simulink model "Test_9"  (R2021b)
settings: Solver=VariableStepAuto  StartTime=0.0  StopTime=180  MaxStep=1/(50*80)
undefined symbols (not defined in the file): Ion, Lithium
libraries: fl_lib x6, nesl_utility x5, spsRMSLib x2, ee_lib x2, spsBatteryLib x1, spsCurrentVoltageSimscapeInterfaceLib x1, simulink x1, spspowerguiLib x1

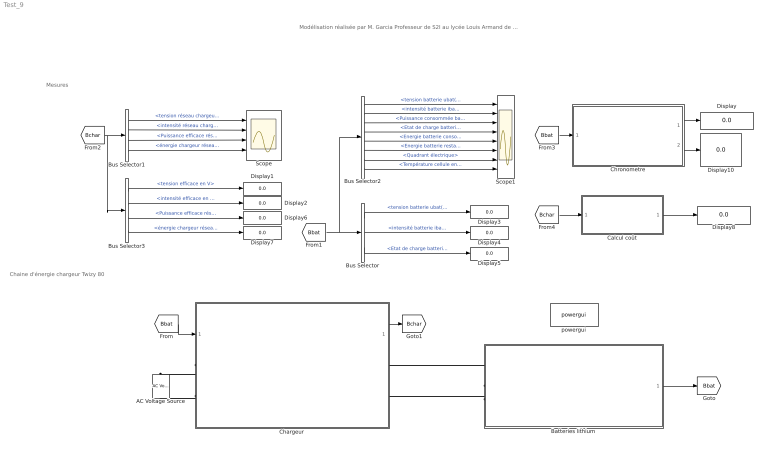
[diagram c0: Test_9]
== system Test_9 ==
  note: Mesures
  note: Chaine d'énergie chargeur Twizy 80
  note: Modélisation réalisée par M. Garcia Professeur de S2I au lycée Louis Armand de Nogent sur Marne
  AC Voltage Source : fl_lib/Electrical/Electrical Sources/AC Voltage Source  amp=230*sqrt(2) V  shift=0 deg  frequency=50 Hz  omega=0 rad/s
  Batteries lithium : Subsystem  mask{Ubat_n=54, Qbat_n=105, Soc_init=10, Soc_min=10, T_amb=35, T_init=35, Nb_cycles=1000, Nb_charge_mensuelle=20, Nb_mois=0}
      mask prompts: Ubat_n "Tension nominale batterie en V"; Qbat_n "Capacité nominale en A.h"; Soc_init "Etat de charge initial"; Soc_min "Seuil minimum en %"; T_amb "Température ambiante extérieure en °C"; T_init "Température initiale du bloc batteries en °C"; Nb_cycles "Durée de vie batterie en nombre de cycles"; Nb_charge_mensuelle "Nombre de recharges mensuelles"; Nb_mois "Nombre de mois d'utilisation"
  Bus Selector : BusSelector  OutputSignals=tension batterie ubat(t),intensité batterie ibat(t),Etat de charge batterie soc(t) en %
  Bus Selector1 : BusSelector  OutputSignals=tension réseau chargeur en V,intensité réseau chargeur en A,Puissance efficace réseau chargeur en W,énergie chargeur réseau en Wh
  Bus Selector2 : BusSelector  OutputSignals=tension batterie ubat(t),intensité batterie ibat(t),Puissance consommée batterie pbat(t) en W,Etat de charge batterie soc(t) en %,Energie batterie consommée wbat_cons(t) en Wh,Energie batterie restante wbat_rest(t) en Wh,Quadrant électrique,Température cellule en °C
  Bus Selector3 : BusSelector  OutputSignals=tension efficace en V,intensité efficace en A,Puissance efficace réseau chargeur en W,énergie chargeur réseau en Wh
  Calcul coût : Subsystem  mask{P_Hc=0.1243}
      mask prompts: P_Hc "Coût du kWh en € TTC"
  Chargeur : Subsystem  mask{Imax=30, rend_charg=94, Fp_charg=0.9, Long=3.75, Se=2.5}
      mask prompts: Imax "Intensité maximale de charge en A"; rend_charg "Rendement chargeur en %"; Fp_charg "Facteur de puissance chargeur"; Long "Longueur câble en m"; Se "Section câble en mm²"
  Chronometre : Subsystem
  Display{,1..8,10} (10 alike) : Display
  Scope : Scope  NumInputPorts=4
  Scope1 : Scope  NumInputPorts=8
  powergui : spspowerguiLib/powergui  Priority=1  SimulationMode=Discrete  SampleTime=0.1  frequency=60  Iterations=50  frequencyindice=0  Pbase=100e6  ErrMax=1e-4  UnitsV=kV  UnitsW=MW  buscounter=0  FunctionMessages=off  echomessages=off  EnableUseOfTLC=off  CurrentSourceSwitches=off  DisableSnubberDevices=off  DisableRonSwitches=off  DisableVfSwitches=off  DisplayEquations=off  AutomaticDiscreteSolvers=on  SolverType=Tustin/Backward Euler (TBE)  Interpol=off  ExternalGateDelay=off  methode=off  Ts=100  x0status=blocks  SPID=on  SwTol=0  HookPort=off  NonlinearTolerance=1e-4  nMaxIteration=100  ContinueOnMaxIteration=off  RestoreLinks=warning  ResistiveCurrentMeasurement=off  Frange=[0:2:500]  Ylog=off  Xlog=on  ShowGrid=off  save=off  variable=ZData  structure=0  ZoomFFT=off  StartTime=0.0  cycles=1  DisplayStyle=1  fundamental=60  FreqAxis=off  MaxFrequency=1000  frequencyindicesteady=1  RmsSteady=1  display=off
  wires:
  Bus Selector/2 -> Display4/1  "<intensité batterie ibat(t)>"
  [Bbat] -> Bus Selector2/1, Bus Selector/1
  Bus Selector2/1 -> Scope1/1  "<tension batterie ubat(t)>"
  Bus Selector2/2 -> Scope1/2  "<intensité batterie ibat(t)>"
  Bus Selector2/3 -> Scope1/3  "<Puissance consommée batterie pbat(t) en W>"
  Bus Selector/1 -> Display3/1  "<tension batterie ubat(t)>"
  Bus Selector/3 -> Display5/1  "<Etat de charge batterie soc(t) en %>"
  Batteries lithium/1(Bus batterie) -> [Bbat]
  Bus Selector2/4 -> Scope1/4  "<Etat de charge batterie soc(t) en %>"
  Bus Selector2/7 -> Scope1/7  "<Quadrant électrique>"
  Bus Selector2/5 -> Scope1/5  "<Energie batterie consommée wbat_cons(t) en Wh>"
  Bus Selector2/6 -> Scope1/6  "<Energie batterie restante wbat_rest(t) en Wh>"
  [Bbat] -> Chargeur/1(bus_bat)
  Chargeur/1(Bus_chargeur) -> [Bchar]
  [Bchar] -> Bus Selector3/1, Bus Selector1/1
  Bus Selector1/1 -> Scope/1  "<tension réseau chargeur en V>"
  Bus Selector1/2 -> Scope/2  "<intensité réseau chargeur en A>"
  Bus Selector1/3 -> Scope/3  "<Puissance efficace réseau chargeur en W>"
  Bus Selector1/4 -> Scope/4  "<énergie chargeur réseau en Wh>"
  Bus Selector3/1 -> Display1/1  "<tension efficace en V>"
  Bus Selector3/2 -> Display2/1  "<intensité efficace en A>"
  Bus Selector3/3 -> Display6/1  "<Puissance efficace réseau chargeur en W>"
  Bus Selector3/4 -> Display7/1  "<énergie chargeur réseau en Wh>"
  [Bbat] -> Chronometre/1(Bus Batterie)
  [Bchar] -> Calcul coût/1(Bus chargeur)
  Calcul coût/1(Cout en €) -> Display8/1
  Chronometre/2(Mesure temps de charge HH mm ss) -> Display10/1
  Chronometre/1(Mesure temps de charge h) -> Display/1
  Bus Selector2/8 -> Scope1/8  "<Température cellule en °C>"
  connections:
  Batteries lithium/LConn1 -- Chargeur/RConn1
  Batteries lithium/LConn2 -- Chargeur/RConn2
  Chargeur/LConn2 -- AC Voltage Source/RConn1
  Chargeur/LConn1 -- AC Voltage Source/LConn1

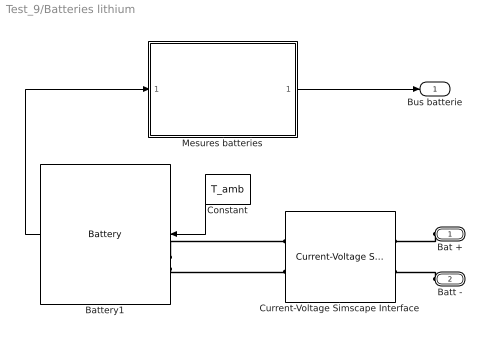
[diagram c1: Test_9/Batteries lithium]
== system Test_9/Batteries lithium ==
  Battery1 : spsBatteryLib/Battery  BatType=Lithium-Ion  ShowTempParam=on  ThermalPreset=no  ShowAgeParam=on  NomV=Ubat_n  NomQ=Qbat_n  SOC=Soc_init  Batt_Tr=30  PresetModel=on  MaxQ=105  MinV=40.5  FullV=62.8553  Dis_rate=45.6522  R=0.0051429  Normal_OP=94.9565  expZone="[58.3408       5.1587]"  current=[100 150 200]  Units=Time  Tci=T_init  NomT=25  T2=0  MaxQ2=Qbat_n/1.1517  FullV2=1.1933*Ubat_n  Normal_OP2=Ubat_n/1.1576  expZone2=[1.1338*Ubat_n Qbat_n/61]  Rca=0.06  ti=1000  Dp=0  Neq0=Nb_charge_mensuelle*Nb_mois  Tsim=30  Ta1=23  Qeol=0.9*Qbat_n  Reol=0.0126*1.2  Char_age=[0.38*Qbat_n, 0.495*Qbat_n]  Dis_age=[0.38*Qbat_n, 2*Qbat_n]  N1=Nb_cycles  N2=7*Nb_cycles  N3=Nb_cycles/1.5  N4=Nb_cycles*0.9733  Ta2=45  N5=Nb_cycles*0.655
  Constant : Constant  Value=T_amb
  Current-Voltage Simscape Interface : spsCurrentVoltageSimscapeInterfaceLib/Current-Voltage Simscape Interface  DFT=off  FMode=Unit delay (discrete)  T=1e-6  Ts=-1  i0=0  v0=52  Sd=Simscape side  Measurements=off
  Mesures batteries : Subsystem
  Bat + : PMIOPort  Side=Left
  Batt - : PMIOPort  Port=2  Side=Left
  Bus batterie : Outport  VectorParamsAs1DForOutWhenUnconnected=off
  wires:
  Battery1/1 -> Mesures batteries/1(Bus batteries)
  Mesures batteries/1(Bus_ batteries) -> Bus batterie/1
  Constant/1 -> Battery1/1
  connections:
  Battery1/LConn2 -- Current-Voltage Simscape Interface/LConn2
  Battery1/LConn1 -- Current-Voltage Simscape Interface/LConn1
  Bat +/RConn1 -- Current-Voltage Simscape Interface/RConn1
  Batt -/RConn1 -- Current-Voltage Simscape Interface/RConn2

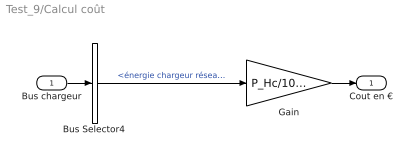
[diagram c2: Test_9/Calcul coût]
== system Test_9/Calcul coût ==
  Bus chargeur : Inport
  Bus Selector4 : BusSelector  OutputSignals=énergie chargeur réseau en Wh
  Gain : Gain  Gain=P_Hc/1000
  Cout en € : Outport  VectorParamsAs1DForOutWhenUnconnected=off
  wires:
  Bus Selector4/1 -> Gain/1  "<énergie chargeur réseau en Wh>"
  Gain/1 -> Cout en €/1
  Bus chargeur/1 -> Bus Selector4/1

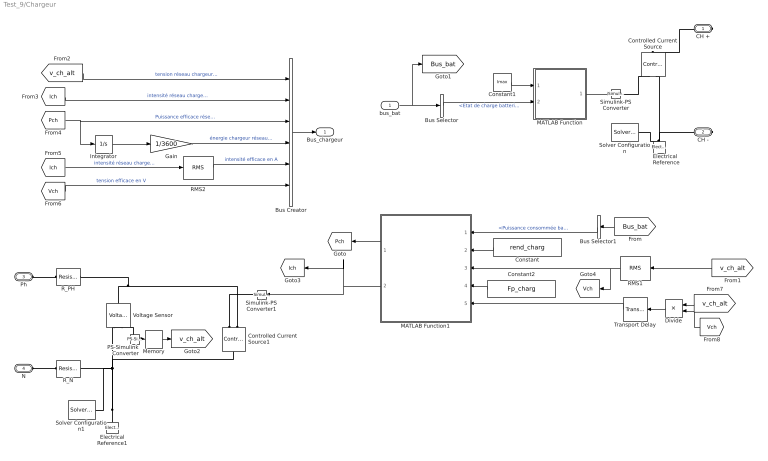
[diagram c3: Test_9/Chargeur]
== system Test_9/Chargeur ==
  bus_bat : Inport
  Bus Creator : BusCreator  Inputs=6
  Bus Selector : BusSelector  OutputSignals=Etat de charge batterie soc(t) en %
  Bus Selector1 : BusSelector  OutputSignals=Puissance consommée batterie pbat(t) en W
  Constant : Constant  Value=rend_charg
  Constant1 : Constant  Value=Imax
  Constant2 : Constant  Value=Fp_charg
  Controlled Current Source : fl_lib/Electrical/Electrical Sources/Controlled Current Source
  Controlled Current Source1 : fl_lib/Electrical/Electrical Sources/Controlled Current Source
  Divide : Product  Inputs=*/
  Electrical Reference : fl_lib/Electrical/Electrical Elements/Electrical Reference
  Electrical Reference1 : fl_lib/Electrical/Electrical Elements/Electrical Reference
  Gain : Gain  Gain=1/3600
  Integrator : Integrator
  MATLAB Function : MATLAB Function  TreatAsAtomicUnit=on
  MATLAB Function1 : MATLAB Function  TreatAsAtomicUnit=on
  Memory : Memory  LinearizeMemory=on
  PS-Simulink Converter : nesl_utility/PS-Simulink Converter  PhysicalDomain=network_engine_domain  SubClassName=ps_output  LeftPortType=input  RightPortType=output  PseudoPeriodic=off  Frequencies=[]  Unit=1  AffineConversion=off
  RMS1 : spsRMSLib/RMS  TrueRMS=on  Freq=50  RMSInit=230  Ts=0
  RMS2 : spsRMSLib/RMS  TrueRMS=on  Freq=50  RMSInit=0  Ts=0
  R_N : ee_lib/Passive/Resistor  R=Long*22e-3/Se Ohm  R_tol=5  enable_R_tol=0  tol_distribution=1  nSigma=4  enable_operating_limits=0  operating_limit_action=2  max_working_voltage=100 V  power_rating=1 W  enable_faults=0  fault_action=1  R_faulted=inf Ohm  enable_temporal_fault=0  t_fault=1 s  enable_behavioral_fault=0  max_permissible_current=1 A  t_fail_on_current=1 s  noise_mode=0  sample_time=1e-3 s  repeatability=1  auto_seed=676943032  user_seed=0  Tdevice=25 degC  power_derating_T1=70 degC  power_derating_T2=155 degC  operating_temperature_range_vec=[-50, 150] degC  alpha=3.93e-3 1/K  Tmeas=25 degC  thermal_mass=100 J/K  temperature_specify=off  temperature_priority=High  temperature=298.15 K  temperature_nominal_specify=off  temperature_nominal_unit=K  temperature_nominal_value=1
  R_PH : ee_lib/Passive/Resistor  R=Long*22e-3/Se Ohm  R_tol=5  enable_R_tol=0  tol_distribution=1  nSigma=4  enable_operating_limits=0  operating_limit_action=2  max_working_voltage=100 V  power_rating=1 W  enable_faults=0  fault_action=1  R_faulted=inf Ohm  enable_temporal_fault=0  t_fault=1 s  enable_behavioral_fault=0  max_permissible_current=1 A  t_fail_on_current=1 s  noise_mode=0  sample_time=1e-3 s  repeatability=1  auto_seed=4168664255  user_seed=0  Tdevice=25 degC  power_derating_T1=70 degC  power_derating_T2=155 degC  operating_temperature_range_vec=[-50, 150] degC  alpha=3.93e-3 1/K  Tmeas=25 degC  thermal_mass=100 J/K  temperature_specify=off  temperature_priority=High  temperature=298.15 K  temperature_nominal_specify=off  temperature_nominal_unit=K  temperature_nominal_value=1
  Simulink-PS Converter : nesl_utility/Simulink-PS Converter  PhysicalDomain=network_engine_domain  SubClassName=ps_input  LeftPortType=input  RightPortType=output  PseudoPeriodic=off  Frequencies=[]  NoiseDistribution=none  NoiseParameters=[]  Unit=A  AffineConversion=off  FilteringAndDerivatives=provide  SimscapeFilterOrder=1  InputFilterTimeConstant=0.001  UdotUserProvided=0
  Simulink-PS Converter1 : nesl_utility/Simulink-PS Converter  PhysicalDomain=network_engine_domain  SubClassName=ps_input  LeftPortType=input  RightPortType=output  PseudoPeriodic=off  Frequencies=[]  NoiseDistribution=none  NoiseParameters=[]  Unit=1  AffineConversion=off  FilteringAndDerivatives=provide  SimscapeFilterOrder=1  InputFilterTimeConstant=0.001  UdotUserProvided=0
  Solver Configuration : nesl_utility/Solver Configuration  PhysicalDomain=network_engine_domain  SubClassName=solver  LeftPortType=input  RightPortType=generic  Tones=[]  Harmonics=[]  SimulateNoise=off  Profile=off  UseLocalSampling=off  EnableSwitchedLinearOptims=on  FrequencyDomain=off  UseCCode=off  RelTol=0.001  AbsTol=1e-06  MinStep=1e-09  ToWorkspace=off  RevertToSquareIcSolve=off  NumHomotopyIterations=100  PhasorMode=off  PhasorModeNumHarmonics=1  DoDC=off  ResidualTolerance=1e-09  UseLocalSolver=off  LocalSolverChoice=NE_BACKWARD_EULER_ADVANCER  LocalSolverSampleTime=0.01  DoFixedCost=off  MaxNonlinIter=3  MaxModeIter=2  ComputeImpulses=off  ImpulseIterations=2  LinearAlgebra=auto  EquationFormulation=NE_TIME_EF  DelaysMemoryBudget=1024  AutomaticFiltering=on  FilteringTimeConstant=0.001  PartitionStorageMethod=AS_NEEDED  PartitionMemoryBudget=1024  PartitionMethod=FAST
  Solver Configuration1 : nesl_utility/Solver Configuration  PhysicalDomain=network_engine_domain  SubClassName=solver  LeftPortType=input  RightPortType=generic  Tones=[]  Harmonics=[]  SimulateNoise=off  Profile=off  UseLocalSampling=off  EnableSwitchedLinearOptims=on  FrequencyDomain=off  UseCCode=off  RelTol=0.001  AbsTol=1e-06  MinStep=1e-09  ToWorkspace=off  RevertToSquareIcSolve=off  NumHomotopyIterations=100  PhasorMode=off  PhasorModeNumHarmonics=1  DoDC=off  ResidualTolerance=1e-09  UseLocalSolver=off  LocalSolverChoice=NE_BACKWARD_EULER_ADVANCER  LocalSolverSampleTime=0.001  DoFixedCost=off  MaxNonlinIter=3  MaxModeIter=2  ComputeImpulses=off  ImpulseIterations=2  LinearAlgebra=auto  EquationFormulation=NE_TIME_EF  DelaysMemoryBudget=1024  AutomaticFiltering=on  FilteringTimeConstant=0.001  PartitionStorageMethod=AS_NEEDED  PartitionMemoryBudget=1024  PartitionMethod=FAST
  Transport Delay : TransportDelay  DelayTime=acos(Fp_charg)*0.02/(2*pi)
  Voltage Sensor : fl_lib/Electrical/Electrical Sensors/Voltage Sensor
  CH + : PMIOPort  Side=Right
  CH - : PMIOPort  Port=2  Side=Right
  Ph : PMIOPort  Port=3  Side=Left
  N : PMIOPort  Port=4  Side=Left
  Bus_chargeur : Outport  VectorParamsAs1DForOutWhenUnconnected=off
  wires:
  bus_bat/1 -> [Bus_bat], Bus Selector/1
  Bus Selector/1 -> MATLAB Function/2(soc)  "<Etat de charge batterie soc(t) en %>"
  Constant/1 -> MATLAB Function1/2(rend_chargeur)
  MATLAB Function/1(Ich) -> Simulink-PS Converter/1
  MATLAB Function1/2(i_ch) -> [Ich], Simulink-PS Converter1/1
  [Bus_bat] -> Bus Selector1/1
  Bus Selector1/1 -> MATLAB Function1/1(P_bat)  "<Puissance consommée batterie pbat(t) en W>"
  [v_ch_alt] -> RMS1/1
  PS-Simulink Converter/1 -> Memory/1
  Memory/1 -> [v_ch_alt]
  MATLAB Function1/1(Pch) -> [Pch]
  [v_ch_alt] -> Bus Creator/1  "tension réseau chargeur en V"
  [Ich] -> Bus Creator/2  "intensité réseau chargeur en A"
  [Pch] -> Integrator/1, Bus Creator/3  "Puissance efficace réseau chargeur en W"
  Gain/1 -> Bus Creator/4  "énergie chargeur réseau en Wh"
  Bus Creator/1 -> Bus_chargeur/1
  Constant1/1 -> MATLAB Function/1(Imax)
  Constant2/1 -> MATLAB Function1/4(Fp_ch)
  Integrator/1 -> Gain/1
  Divide/1 -> Transport Delay/1
  RMS1/1 -> [Vch], MATLAB Function1/3(Vch)
  [Ich] -> RMS2/1  "intensité réseau chargeur en A"
  RMS2/1 -> Bus Creator/5  "intensité efficace en A"
  [Vch] -> Bus Creator/6  "tension efficace en V"
  [v_ch_alt] -> Divide/1
  [Vch] -> Divide/2
  Transport Delay/1 -> MATLAB Function1/5(sinus)
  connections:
  Electrical Reference/LConn1 -- Solver Configuration/RConn1 -- Controlled Current Source/RConn2 -- CH -/RConn1
  CH +/RConn1 -- Controlled Current Source/LConn1
  Simulink-PS Converter/RConn1 -- Controlled Current Source/RConn1
  R_PH/LConn1 -- Ph/RConn1
  Electrical Reference1/LConn1 -- Solver Configuration1/RConn1 -- R_N/RConn1 -- Controlled Current Source1/LConn1 -- Voltage Sensor/RConn2
  Controlled Current Source1/RConn1 -- Simulink-PS Converter1/RConn1
  PS-Simulink Converter/LConn1 -- Voltage Sensor/RConn1
  Controlled Current Source1/RConn2 -- Voltage Sensor/LConn1 -- R_PH/RConn1
  N/RConn1 -- R_N/LConn1

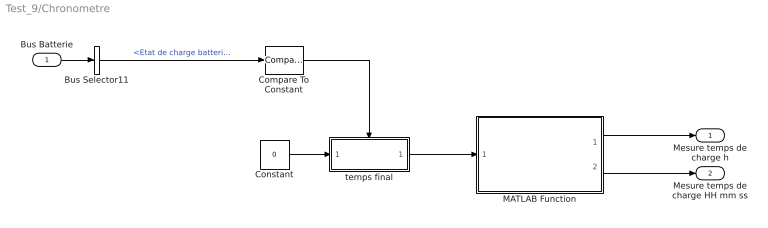
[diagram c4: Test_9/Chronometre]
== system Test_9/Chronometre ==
  Bus Batterie : Inport
  Bus Selector11 : BusSelector  OutputSignals=Etat de charge batterie soc(t) en %
  Compare To Constant : simulink/Logic and Bit Operations/Compare To Constant  relop=<  const=100  OutDataTypeStr=boolean
  Constant : Constant  Value=0
  MATLAB Function : MATLAB Function  TreatAsAtomicUnit=on
  temps final : Subsystem
  Mesure temps de charge h : Outport  VectorParamsAs1DForOutWhenUnconnected=off
  Mesure temps de charge HH mm ss : Outport  Port=2  VectorParamsAs1DForOutWhenUnconnected=off
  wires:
  Compare To Constant/1 -> temps final/Enable
  Bus Selector11/1 -> Compare To Constant/1  "<Etat de charge batterie soc(t) en %>"
  Bus Batterie/1 -> Bus Selector11/1
  Constant/1 -> temps final/1(tps_init)
  temps final/1(delta_tps) -> MATLAB Function/1(u)
  MATLAB Function/2(HH_M_SS) -> Mesure temps de charge HH mm ss/1
  MATLAB Function/1(dec) -> Mesure temps de charge h/1

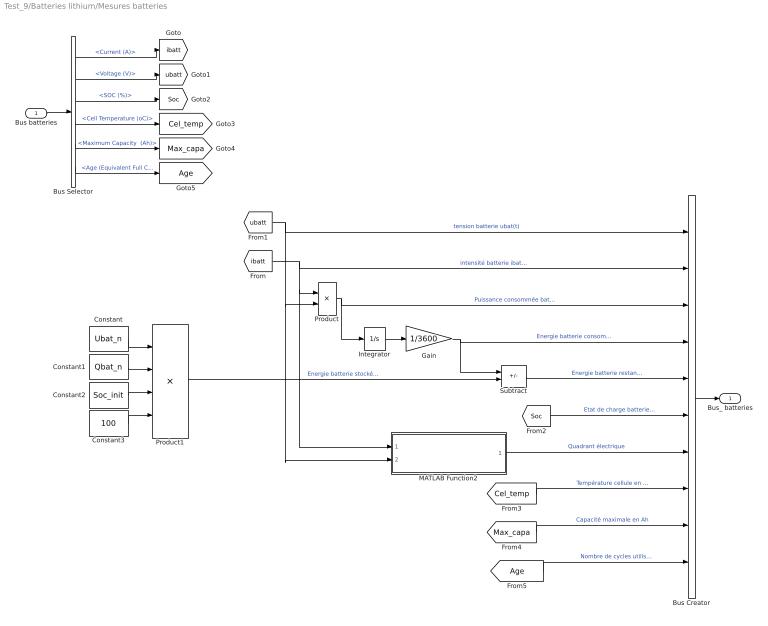
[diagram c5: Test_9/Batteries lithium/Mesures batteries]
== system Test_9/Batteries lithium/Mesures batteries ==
  Bus batteries : Inport
  Bus Creator : BusCreator  Inputs=10
  Bus Selector : BusSelector  OutputSignals="Current (A),Voltage (V),SOC (%),Cell Temperature (oC),Maximum Capacity  (Ah),Age (Equivalent Full Cycles)"
  Constant : Constant  Value=Ubat_n
  Constant1 : Constant  Value=Qbat_n
  Constant2 : Constant  Value=Soc_init
  Constant3 : Constant  Value=100
  Gain : Gain  Gain=1/3600
  Integrator : Integrator
  MATLAB Function2 : MATLAB Function  TreatAsAtomicUnit=on
  Product : Product
  Product1 : Product  Inputs=***/
  Subtract : Sum  Inputs=-+
  Bus_ batteries : Outport  VectorParamsAs1DForOutWhenUnconnected=off
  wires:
  Bus batteries/1 -> Bus Selector/1
  Product/1 -> Bus Creator/3, Integrator/1  "Puissance consommée batterie pbat(t) en W"
  Bus Creator/1 -> Bus_ batteries/1
  Integrator/1 -> Gain/1
  Gain/1 -> Bus Creator/4, Subtract/1  "Energie batterie consommée wbat_cons(t) en Wh"
  [ibatt] -> Bus Creator/2, MATLAB Function2/1(I_bat), Product/1  "intensité batterie ibat(t)"
  Bus Selector/1 -> [ibatt]  "<Current (A)>"
  Bus Selector/2 -> [ubatt]  "<Voltage (V)>"
  [ubatt] -> MATLAB Function2/2(U_bat), Product/2, Bus Creator/1  "tension batterie ubat(t)"
  Bus Selector/3 -> [Soc]  "<SOC (%)>"
  [Soc] -> Bus Creator/6  "Etat de charge batterie soc(t) en %"
  MATLAB Function2/1(Quadrant_elec) -> Bus Creator/7  "Quadrant électrique"
  Constant/1 -> Product1/1
  Constant1/1 -> Product1/2
  Constant2/1 -> Product1/3
  Constant3/1 -> Product1/4
  Subtract/1 -> Bus Creator/5  "Energie batterie restante wbat_rest(t) en Wh"
  Product1/1 -> Subtract/2  "Energie batterie stockée wstock_batt(t) en Wh"
  Bus Selector/4 -> [Cel_temp]  "<Cell Temperature (oC)>"
  Bus Selector/5 -> [Max_capa]  "<Maximum Capacity  (Ah)>"
  Bus Selector/6 -> [Age]  "<Age (Equivalent Full Cycles)>"
  [Cel_temp] -> Bus Creator/8  "Température cellule en °C"
  [Max_capa] -> Bus Creator/9  "Capacité maximale en Ah"
  [Age] -> Bus Creator/10  "Nombre de cycles utilisés"

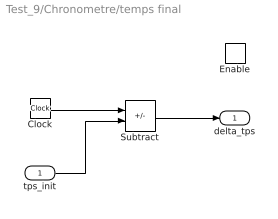
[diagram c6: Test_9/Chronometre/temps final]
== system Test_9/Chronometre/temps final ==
  tps_init : Inport
  Enable : EnablePort
  Clock : Clock
  Subtract : Sum  Inputs=+-
  delta_tps : Outport  VectorParamsAs1DForOutWhenUnconnected=off
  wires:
  Clock/1 -> Subtract/1
  tps_init/1 -> Subtract/2
  Subtract/1 -> delta_tps/1

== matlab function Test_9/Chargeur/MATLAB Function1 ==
function [Pch,i_ch]= fcn(P_bat,rend_chargeur,Vch,Fp_ch,sinus)
Pch = -P_bat/(rend_chargeur/100);
I_alt_ch = Pch/(Vch*Fp_ch);
i_ch=I_alt_ch*sinus;
end

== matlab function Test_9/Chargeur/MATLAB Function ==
function Ich = fcn(Imax,soc)
if soc < 100
Ich = Imax;
else
Ich=0;
end
end

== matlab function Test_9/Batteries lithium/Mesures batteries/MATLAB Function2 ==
function Quadrant_elec = fcn(I_bat,U_bat)
if U_bat > 0.8
    if I_bat > 0.3
        Quadrant_elec = 1;
    elseif I_bat < -0.5
        Quadrant_elec = 4;
    else
        Quadrant_elec = 0;
    end
elseif U_bat < -0.8
    if I_bat > 0.5
        Quadrant_elec = 2;
    elseif I_bat < -0.5
        Quadrant_elec = 3;
    else
        Quadrant_elec = 0;
    end
else
    Quadrant_elec = 0;
end
end

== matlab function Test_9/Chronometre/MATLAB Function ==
function [dec,HH_M_SS]= fcn(u)
dec=u/3600;
hour = floor(dec);
min=floor((dec-hour)*60);
sec=floor(rem((dec-hour)*60,1)*60);
HH_M_SS=[hour,min,sec];
end
